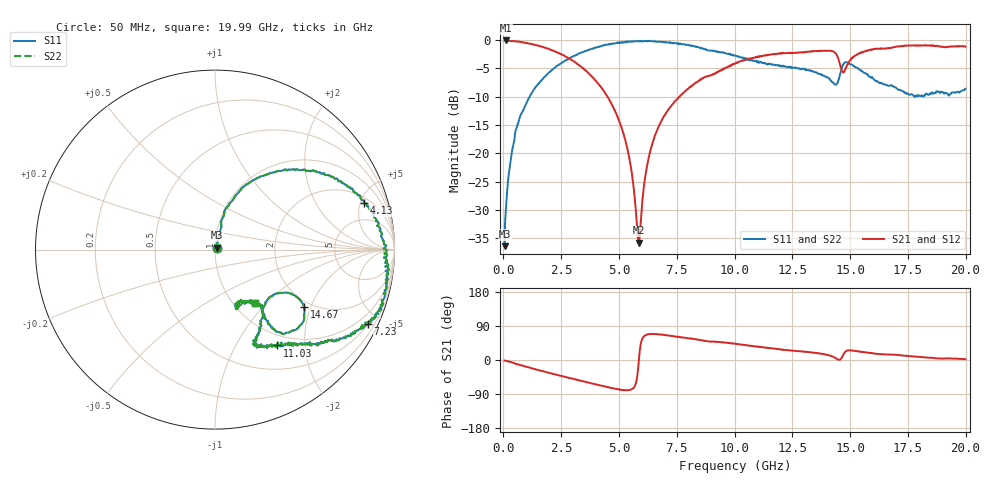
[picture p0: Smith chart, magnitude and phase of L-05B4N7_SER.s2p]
! Data Taken on a HP 8720C VNA using a series-through fixture with TRL* de-embedding
#	mhz	s	ma	r	50
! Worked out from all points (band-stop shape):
!   998 points, 50 MHz to 19.99 GHz, reference 50 ohm
!   highest |S21| = -0.08 dB at 90 MHz (marker M1); lowest = -35.8 dB at 5.85 GHz (marker M2)
!   |S21| within 3 dB of the highest: 10.9 GHz to 14.48 GHz (3.573 GHz wide, 28.2 % of centre); 15.11 GHz to end of sweep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
!   lowest |S11| = -36.4 dB at 50 MHz (marker M3), VSWR 1.03, Z = 51 + j1.14 ohm
!   |S11| at or under -10 dB: start of sweep to 1.128 GHz; 17.76644 GHz to 17.79591 GHz (29.47 MHz wide, 0.166 % of centre); 17.84853 GHz to 17.85327 GHz (4.74 MHz wide, 0.0266 % of centre)
!   |S22| runs from -36.4 to -0.1 dB; largest |S21 - S12| = 0
!   S11 on the Smith chart (normalised r, x): 50 MHz: 1.02, +0.02; 4.13 GHz: 2.55, +5.45; 7.23 GHz: 0.51, -4.27; 11.03 GHz: 0.83, -1.50; 14.67 GHz: 1.83, -1.81; 19.99 GHz: 1.25, -0.86
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50  0.01515 47.5  0.9891 -1.4  0.9891 -1.4  0.01515 47.5
90  0.02874 70.0  0.9907 -1.9  0.9907 -1.9  0.02874 70.0
330  0.09271 72.8  0.9785 -5.7  0.9785 -5.7  0.09271 72.8
790  0.2274 76.0  0.9573 -14.5  0.9573 -14.5  0.2274 76.0
2090  0.541 52.8  0.8112 -35.6  0.8112 -35.6  0.541 52.8
3390  0.7756 30.6  0.5748 -55.6  0.5748 -55.6  0.7756 30.6
4130  0.8714 17.2  0.4042 -66.5  0.4042 -66.5  0.8714 17.2
5270  0.9686 -5.1  0.1319 -79.9  0.1319 -79.9  0.9686 -5.1
5550  0.9778 -9.8  0.06824 -77.1  0.06824 -77.1  0.9778 -9.8
5850  0.972 -13.6  0.01622 -7.3  0.01622 -7.3  0.972 -13.6
6210  0.9737 -18.6  0.07674 66.8  0.07674 66.8  0.9737 -18.6
6710  0.9669 -22.5  0.1712 67.9  0.1712 67.9  0.9669 -22.5
7230  0.9488 -26.0  0.2579 63.4  0.2579 63.4  0.9488 -26.0
10030  0.7293 -46.3  0.6231 43.0  0.6231 43.0  0.7293 -46.3
11030  0.636 -57.1  0.7095 34.8  0.7095 34.8  0.636 -57.1
13350  0.5299 -63.4  0.7904 19.6  0.7904 19.6  0.5299 -63.4
14290  0.416 -48.4  0.7908 7.7  0.7908 7.7  0.416 -48.4
14670  0.5919 -32.8  0.525 9.5  0.525 9.5  0.5919 -32.8
15050  0.6079 -50.5  0.6882 25.0  0.6882 25.0  0.6079 -50.5
16670  0.3942 -50.6  0.8452 14.5  0.8452 14.5  0.3942 -50.6
18670  0.3397 -70.4  0.8828 4.5  0.8828 4.5  0.3397 -70.4
19990  0.3707 -52.7  0.8746 2.2  0.8746 2.2  0.3707 -52.7
